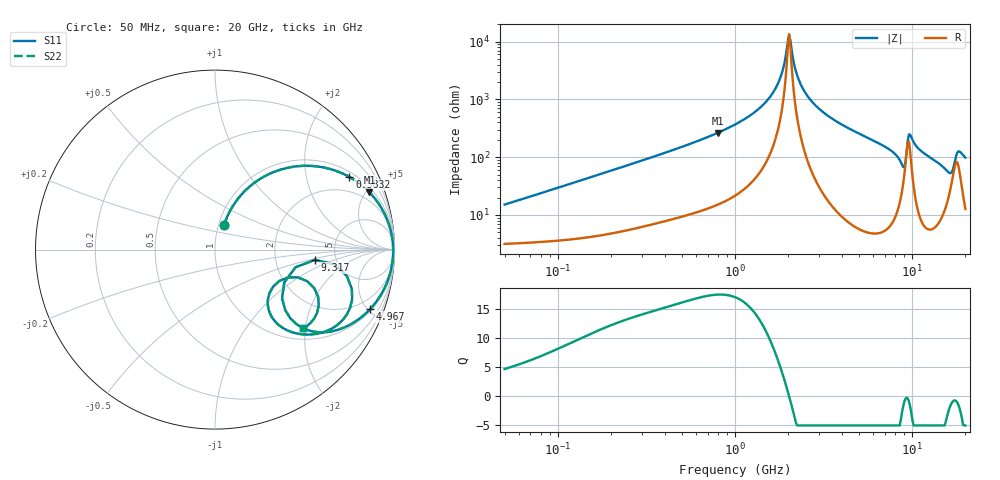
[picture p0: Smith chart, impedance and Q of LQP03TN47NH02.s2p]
!Murata Part Number: LQP03TN47NH02
!These Parameters are Measured in Series Mode Connection
!  o--[Z]--o
!Port1  Port2
!  o-------o
!Freq. Start=50[MHz] Stop=20[GHz], 401[Steps]
# Hz S RI R 50
!Freq.(Hz) S11(Real) S11(Imag) S21(Real) S21(Imag) S12(Real) S12(Imag) S22(Real) S22(Imag)
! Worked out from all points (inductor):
!   401 points, 50 MHz to 20 GHz, reference 50 ohm
!   read as one part in series: L = 46.8 nH near 51.52 MHz
!   highest Q = 17.5 at 798.8 MHz (marker M1), where L = 52.5 nH
!   self-resonance near 1.992 GHz
!   S11 on the Smith chart (normalised r, x): 50 MHz: 1.06, +0.30; 583.2 MHz: 1.21, +3.57; 4.967 GHz: 1.12, -5.19; 9.317 GHz: 3.45, -0.57; 20 GHz: 1.25, -1.95
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5e7  0.05 0.1363  0.95 -0.1363  0.95 -0.1363  0.05 0.1363
1.364002e8  0.1615 0.3217  0.8385 -0.3217  0.8385 -0.3217  0.1615 0.3217
3.721004e8  0.5435 0.4658  0.4565 -0.4658  0.4565 -0.4658  0.5435 0.4658
5.831961e8  0.7489 0.4048  0.2511 -0.4048  0.2511 -0.4048  0.7489 0.4048
7.987718e8  0.8607 0.3189  0.1393 -0.3189  0.1393 -0.3189  0.8607 0.3189
1e9  0.9185 0.2459  0.0815 -0.2459  0.0815 -0.2459  0.9185 0.2459
1.614971e9  0.9846 0.0794  0.0154 -0.0794  0.0154 -0.0794  0.9846 0.0794
1.820564e9  0.9905 0.0371  0.00946 -0.0371  0.00946 -0.0371  0.9905 0.0371
2.021818e9  0.9925 -5.7e-07  0.00745 5.7e-07  0.00745 5.7e-07  0.9925 -5.7e-07
2.279204e9  0.9912 -0.0427  0.00877 0.0427  0.00877 0.0427  0.9912 -0.0427
2.728004e9  0.9817 -0.1076  0.0183 0.1076  0.0183 0.1076  0.9817 -0.1076
4.966507e9  0.8654 -0.3304  0.1346 0.3304  0.1346 0.3304  0.8654 -0.3304
7.442007e9  0.6431 -0.4568  0.3569 0.4568  0.3569 0.4568  0.6431 -0.4568
8.264682e9  0.5099 -0.446  0.4901 0.446  0.4901 0.446  0.5099 -0.446
8.774992e9  0.3912 -0.3374  0.6088 0.3374  0.6088 0.3374  0.3912 -0.3374
9.316812e9  0.558 -0.0571  0.442 0.0571  0.442 0.0571  0.558 -0.0571
9.892087e9  0.7638 -0.28  0.2362 0.28  0.2362 0.28  0.7638 -0.28
1.131968e10  0.6059 -0.4592  0.3941 0.4592  0.3941 0.4592  0.6059 -0.4592
1.573793e10  0.2996 -0.3369  0.7004 0.3369  0.7004 0.3369  0.2996 -0.3369
1.721783e10  0.4062 -0.1551  0.5938 0.1551  0.5938 0.1551  0.4062 -0.1551
1.828096e10  0.5745 -0.2636  0.4255 0.2636  0.4255 0.2636  0.5745 -0.2636
2e10  0.4917 -0.4392  0.5083 0.4392  0.5083 0.4392  0.4917 -0.4392
